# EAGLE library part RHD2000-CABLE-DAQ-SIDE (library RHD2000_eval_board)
Omnetics PZN-12-AA RHD2000 socket - DAQ side
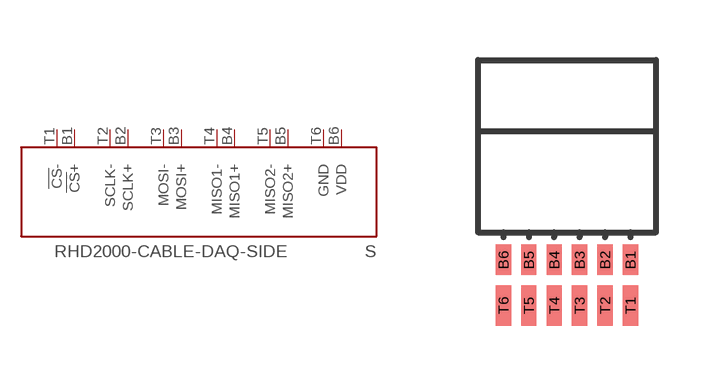
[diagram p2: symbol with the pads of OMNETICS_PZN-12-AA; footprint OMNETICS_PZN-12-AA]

Designator prefix S

## RHD2000-CABLE-DAQ-SIDE  [OMNETICS_PZN-12-AA]
B1  !CS!+
B2  SCLK+
B3  MOSI+
B4  MISO1+
B5  MISO2+
B6  VDD
T1  !CS!-
T2  SCLK-
T3  MOSI-
T4  MISO1-
T5  MISO2-
T6  GND  pwr

## Footprint OMNETICS_PZN-12-AA (pad centres in mm)
smd 0.381 x 0.762: B1 1.587,-1.016; B2 0.953,-1.016; B3 0.318,-1.016; B4 -0.318,-1.016; B5 -0.953,-1.016; B6 -1.587,-1.016
smd 0.381 x 1.016: T1 1.587,-2.159; T2 0.953,-2.159; T3 0.318,-2.159; T4 -0.318,-2.159; T5 -0.953,-2.159; T6 -1.587,-2.159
